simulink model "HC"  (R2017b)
settings: Solver=ode15s  StartTime=0.0  StopTime=1000  RelTol=1e-3
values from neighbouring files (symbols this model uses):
  F_in = F_in/3600    [casADi_CFU.m]    (also in CFU_model_sim.m; CFU_model_sim1.m; run_hc.m = 0.0277777777778; casADi_HC.m = D_hc(1))
  x0 = 2*ones(3*n_x*n_r,1)    [run_hc.m]    (also in RTO.m = X_sol; SS.m = X_sol)
undefined symbols (not defined in the file or in its folder): HC_model_sim
libraries: simulink x1

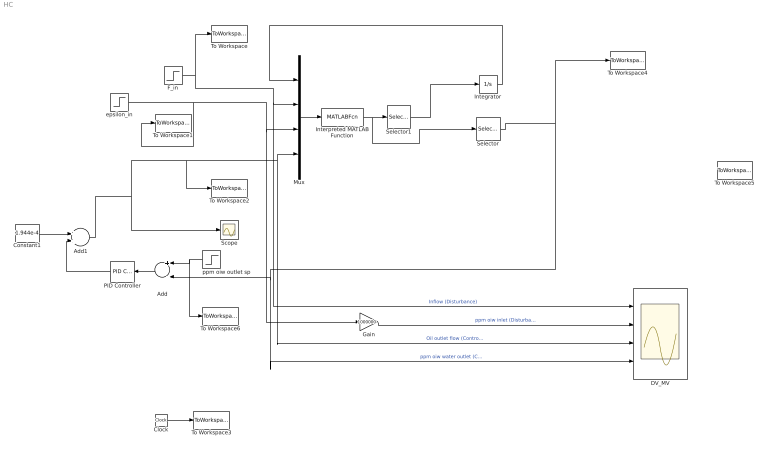
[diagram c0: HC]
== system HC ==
  Add : Sum  Inputs=+-
  Add1 : Sum
  Clock : Clock
  Constant1 : Constant  Value=1.944e-4
  DV_MV : Scope  NumInputPorts=4
  F_in : Step  Time=100  Before=F_in  After=F_in-3/3600  SampleTime=0
  Gain : Gain  Gain=1000000
  Integrator : Integrator  InitialCondition=x0
  Interpreted MATLAB Function : MATLABFcn  MATLABFcn=HC_model_sim(u(1:432),u(433),u(434),u(435))
  Mux : Mux
  PID Controller : simulink/Continuous/PID Controller  Controller=PI  TimeDomain=Continuous-time  SampleTime=-1  IntegratorMethod=Forward Euler  FilterMethod=Forward Euler  Form=Ideal  UseFilter=on  ControllerParametersSource=internal  P=-4.8e-6  I=0.25  D=0  N=100  InitialConditionSource=internal  InitialConditionForIntegrator=0  InitialConditionForFilter=0  ExternalReset=none  LimitOutput=off  UpperSaturationLimit=4*0.6e-6  LowerSaturationLimit=-1.65e-6  LinearizeAsGain=on  AntiWindupMode=clamping  Kb=1  TrackingMode=off  Kt=1  PParamMin=[]  PParamMax=[]  IParamMin=[]  IParamMax=[]  DParamMin=[]  DParamMax=[]  NParamMin=[]  NParamMax=[]  KbParamMin=[]  KbParamMax=[]  KtParamMin=[]  KtParamMax=[]  POutMin=[]  POutMax=[]  IOutMin=[]  IOutMax=[]  DOutMin=[]  DOutMax=[]  NOutMin=[]  NOutMax=[]  KbOutMin=[]  KbOutMax=[]  KtOutMin=[]  KtOutMax=[]  IntegratorOutMin=[]  IntegratorOutMax=[]  FilterOutMin=[]  FilterOutMax=[]  SumOutMin=[]  SumOutMax=[]  SumI1OutMin=[]  SumI1OutMax=[]  SumI2OutMin=[]  SumI2OutMax=[]  SumI3OutMin=[]  SumI3OutMax=[]  SumDOutMin=[]  SumDOutMax=[]  SaturationOutMin=[]  SaturationOutMax=[]  IntegratorContinuousStateAttributes=''  IntegratorStateMustResolveToSignalObject=off  IntegratorRTWStateStorageClass=Auto  FilterContinuousStateAttributes=''  FilterStateMustResolveToSignalObject=off  FilterRTWStateStorageClass=Auto  DifferentiatorICPrevScaledInput=0  DifferentiatorOutMin=[]  DifferentiatorOutMax=[]  InitialConditionSetting=State (most efficient)  FilterDiffOutCoefMin=[]  FilterDiffOutCoefMax=[]  SumDenOutMin=[]  SumDenOutMax=[]  SumNumOutMin=[]  SumNumOutMax=[]  ReciprocalOutMin=[]  ReciprocalOutMax=[]  DivideOutMin=[]  DivideOutMax=[]  TunerSelectOption=Transfer Function Based (PID Tuner App)
  Scope : Scope
  Selector : Selector  InputPortWidth=435  IndexOptions=Index vector (dialog)  Indices=[435]  OutputSizes=1
  Selector1 : Selector  InputPortWidth=435  IndexOptions=Index vector (dialog)  Indices=[1:432]  OutputSizes=1
  To Workspace : ToWorkspace  VariableName=F_in_sim  SampleTime=-1
  To Workspace1 : ToWorkspace  VariableName=e_in_sim  SampleTime=-1
  To Workspace2 : ToWorkspace  VariableName=F_over_sim  SampleTime=-1
  To Workspace3 : ToWorkspace  VariableName=t_sim  SampleTime=-1
  To Workspace4 : ToWorkspace  VariableName=e_out_sim  SampleTime=-1
  To Workspace5 : ToWorkspace  VariableName=OSE_sim  SampleTime=-1
  To Workspace6 : ToWorkspace  VariableName=e_sp_sim  SampleTime=-1
  epsilon_in : Step  Time=600  Before=1500e-6  After=1250e-6  SampleTime=0
  "ppm oiw outlet sp " : Step  Time=400  Before=120  After=120  SampleTime=0
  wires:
  epsilon_in/1 -> To Workspace1/1, Mux/3, Gain/1
  F_in/1 -> To Workspace/1, DV_MV/1, Mux/2  "Inflow (Disturbance)"
  Interpreted MATLAB Function/1 -> Selector/1, Selector1/1
  Integrator/1 -> Mux/1
  Mux/1 -> Interpreted MATLAB Function/1
  Clock/1 -> To Workspace3/1
  Selector/1 -> To Workspace4/1, DV_MV/4, Add/2  "ppm oiw water outlet (CV)"
  Selector1/1 -> Integrator/1
  Gain/1 -> DV_MV/2  "ppm oiw inlet (Disturbance)"
  "ppm oiw outlet sp "/1 -> To Workspace6/1, Add/1
  Add/1 -> PID Controller/1
  Constant1/1 -> Add1/1
  PID Controller/1 -> Add1/2
  Add1/1 -> To Workspace2/1, DV_MV/3, Mux/4, Scope/1  "Oil outlet flow (Control input)"
